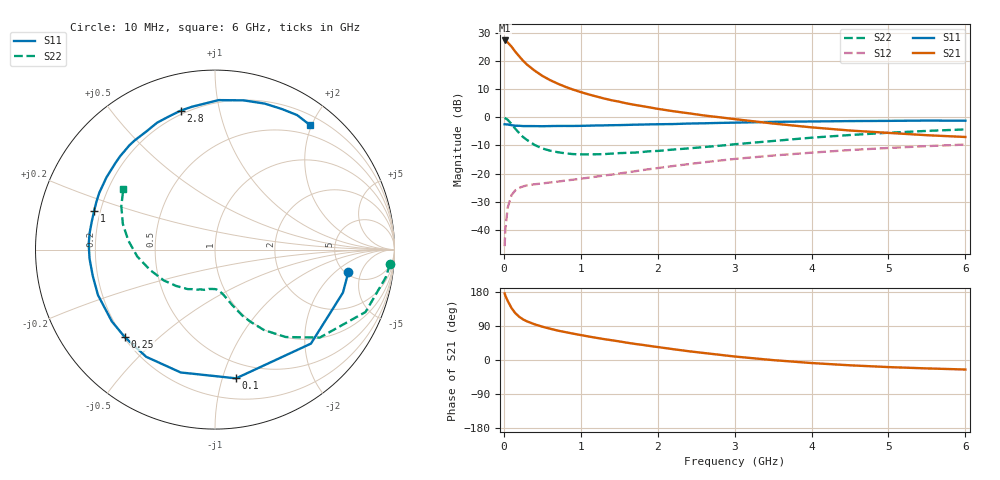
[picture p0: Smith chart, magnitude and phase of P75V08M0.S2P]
! SIEMENS Small Signal Semiconductors
! BFP196
! Si NPN RF Bipolar Junction Transistor in SOT143
! VCE = 5 V  IC = 8 mA
! Common Emitter S-Parameters:  May  1996
# GHz  S  MA  R  50
!  f  S11  S21  S12  S22
! GHz  MAG  ANG  MAG  ANG  MAG  ANG  MAG  ANG
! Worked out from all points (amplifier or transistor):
!   36 points, 10 MHz to 6 GHz, reference 50 ohm
!   highest |S21| = 27.4 dB at 10 MHz (marker M1)
!   |S21| within 3 dB of that: start of sweep to 121.5 MHz
!   unconditionally stable (mu >= 1): 964 MHz to 3.226 GHz
!   at 250 MHz: K = 0.34, MSG = 22.4 dB, |S12| = -24.6 dB
!   at 1.4 GHz: K = 1.14, MAG = 11.0 dB, |S12| = -20.4 dB
!   at 6 GHz: K = 0.98, MSG = 1.3 dB, |S12| = -9.7 dB
!   S11 on the Smith chart (normalised r, x): 10 MHz: 5.31, -3.06; 100 MHz: 0.36, -1.11; 250 MHz: 0.20, -0.39; 1 GHz: 0.18, +0.15; 2.8 GHz: 0.18, +0.77; 6 GHz: 0.34, +1.97
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0.01  0.7537 -9.5  23.43 175.8  0.0051 87.6  0.9786 -4.8
0.02  0.7521 -18.6  22.84 169.7  0.0104 82.3  0.9634 -9.3
0.05  0.7484 -44.4  21.59 156.0  0.0247 68.9  0.908 -22.5
0.1  0.7268 -80.7  18.18 137.1  0.0414 53.2  0.7625 -40.0
0.15  0.7107 -105.6  14.7 123.4  0.0505 43.6  0.6269 -51.0
0.2  0.7097 -122.7  12.24 114.1  0.0557 37.6  0.5241 -58.7
0.25  0.7002 -135.7  10.19 107.1  0.059 34.2  0.447 -63.9
0.3  0.7004 -145.1  8.751 102.0  0.0616 32.0  0.3974 -67.5
0.4  0.6995 -158.8  6.81 94.2  0.0645 29.9  0.3234 -72.8
0.5  0.6967 -167.9  5.494 87.9  0.0667 29.8  0.2798 -76.5
0.6  0.7008 -175.9  4.617 82.6  0.0694 30.6  0.2558 -79.5
0.7  0.7043 177.6  3.993 77.6  0.0718 31.4  0.2403 -82.2
0.8  0.7046 172.4  3.502 73.6  0.075 32.6  0.2293 -85.1
1  0.707 162.3  2.821 65.8  0.081 35.4  0.2199 -90.4
1.1  0.7121 158.2  2.573 62.1  0.0844 36.6  0.2198 -93.2
1.6  0.7349 139.2  1.771 45.7  0.1051 40.7  0.2339 -107.4
2.2  0.7611 120.2  1.29 28.6  0.1362 41.4  0.2675 -124.6
2.8  0.7974 103.9  1.007 13.9  0.1702 38.3  0.3123 -143.2
3.5  0.8332 88.6  0.778 -0.3  0.2094 31.8  0.3802 -162.8
4.5  0.8593 71.2  0.584 -14.0  0.2624 21.0  0.4857 174.0
5.5  0.878 58.6  0.482 -22.2  0.308 9.5  0.575 155.2
6  0.8728 52.8  0.448 -25.1  0.3285 3.1  0.6115 146.7
